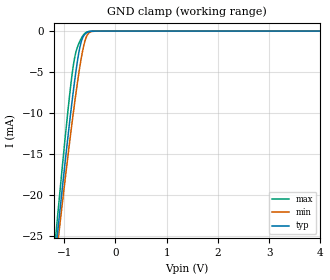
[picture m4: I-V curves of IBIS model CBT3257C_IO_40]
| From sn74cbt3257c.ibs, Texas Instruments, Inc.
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[Model]   CBT3257C_IO_40
Model_type  Terminator
| variable   typ   min   max
C_comp   8.36pF   6.78pF   13.02pF
| C_tri-state   8.36pF   6.78pF   13.02pF
[Temperature Range]   40   100   -40
| Ambient temperature   25   85   -40
[Voltage range]   4   4   4
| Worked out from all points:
|   GND clamp passes 1 mA (typ) near -0.65 V on its own axis
[GND Clamp]
| CBT3257C_IO_40
|   Voltage   I(typ)   I(min)   I(max)
-5V       -286.9mA   -267.5mA   -309.2mA
-1.175V   -27.56mA   -28.75mA   -25.86mA
-1.14V    -25.44mA   -26.81mA   -23.51mA
-1.105V   -23.33mA   -24.88mA   -21.17mA
-1.075V   -21.55mA   -23.24mA   -19.19mA
-920mV    -12.64mA   -15mA      -9.438mA
-815mV    -7.1mA     -9.758mA   -4.012mA
-685mV    -1.8mA     -4.052mA   -1.138mA
-610mV    -508.2uA   -1.614mA   -383.4uA
-550mV    -165.1uA   -514.6uA   -102.8uA
-405mV    -8.507uA   -19.17uA   -1.002uA
4V        495pA      1.539nA    195pA
